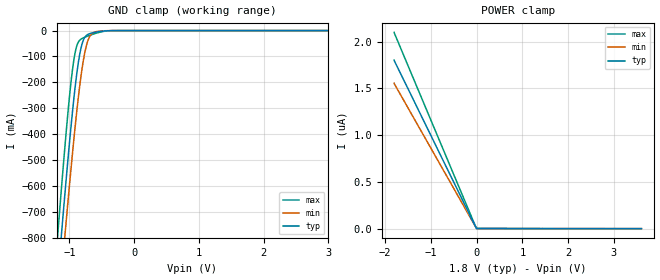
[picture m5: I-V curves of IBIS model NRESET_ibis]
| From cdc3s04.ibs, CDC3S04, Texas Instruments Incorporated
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[Model]   NRESET_ibis
Model_type   Input
Vinl = 630.000mV
Vinh = 1.170V
|   typ   min   max
C_comp   839.5fF   822.7fF   858.5fF
[Voltage Range]   1.800V   1.650V   1.950V
[Temperature Range]   32.0   85.0   -40.0
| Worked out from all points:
|   GND clamp passes 1 mA (typ) near -0.43 V on its own axis
[GND Clamp]
|   Voltage   I(typ)   I(min)   I(max)
-1.8V     -2.926A    -3.001A    -2.86A
-1.192V   -994.5mA   -1.145A    -824.8mA
-1.173V   -934.9mA   -1.088A    -762.6mA
-1.129V   -803mA     -960.3mA   -625.3mA
-1.088V   -681.5mA   -842.2mA   -500.1mA
-1.055V   -588mA     -750.6mA   -405.3mA
-974.5mV  -366.7mA   -529.5mA   -195mA
-917.8mV  -230mA     -384.8mA   -92.21mA
-821.9mV  -67.73mA   -176mA     -33.07mA
-719.3mV  -15.33mA   -41.56mA   -21.34mA
-451.4mV  -1.281mA   -681.2uA   -2.378mA
3.599V    0A         0A         0A
[POWER Clamp]
|   Voltage   I(typ)   I(min)   I(max)
-1.8V     1.802uA    1.555uA    2.099uA
-31.5mV   29.12nA    26.71nA    33.04nA
0V        437.9pA    585.7fA    3.753nA
3.599V    -6pA       0A         -204.8pA
